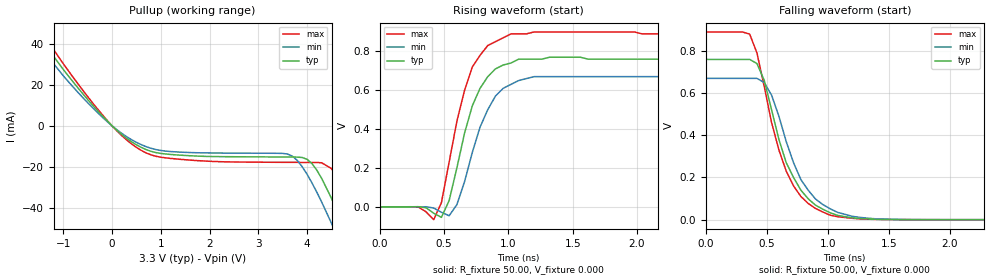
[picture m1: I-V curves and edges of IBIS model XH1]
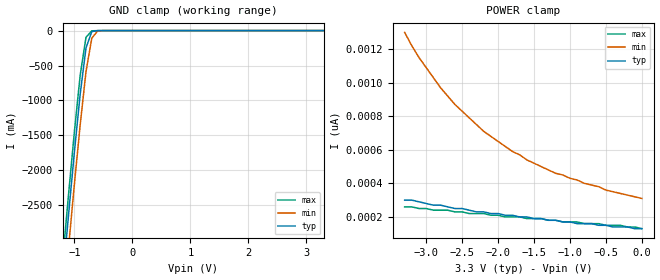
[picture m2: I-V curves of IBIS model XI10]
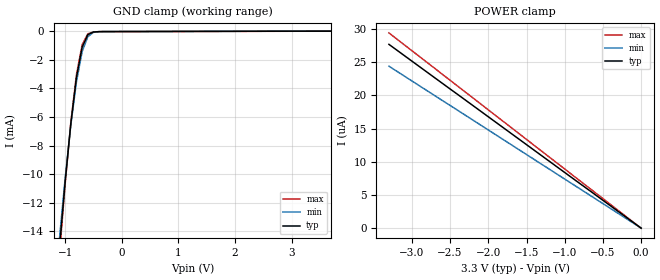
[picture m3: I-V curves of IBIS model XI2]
|   * 9db401d.ibs * IBIS 2.1 Model file
| Rev History
| Rev No.   Description
| 1.0   Initial release
| 1.1   Updated Parasitic Parameters,
|   Input and output C_comp min / Max tightened + Added pin RLC
| 1.2   Update parameters   August 8, 2005
| 1.3   Update XH1, XIO3 Jan. 06, 2010
| 1.4   Add Vmeas, Vref, Ref. May 2010 lp
[IBIS Ver]   2.1
[Comment char]  |_char
[File name]   9db401d.ibs
[Date]   May 10, 2010
[File Rev]   1.4
[Source]   Originated at Integrated Circuit Systems, Inc.
[Disclaimer] (C) Copyright Integrated Circuit Systems, Inc. 2004
   All rights reserved
ICS hereby grants the user of this IBIS model a non-exclusive,
nontransferable license to use this IBIS model under the following terms.
Before using this IBIS model, the user should read this license.
If the user does not accept these terms,  the IBIS model should be
returned to ICS within 30 days.
   The user is granted this license only to use the IBIS model and
is not granted rights to sell, load, rent, lease or license the IBIS
model in whole or in part, or in modified form to anyone other than
user. User may modify the IBIS model to suit its specific
applications but rights to derivative works and such modifications
shall belong to ICS.
   This IBIS model is provided on an "AS IS" basis and ICS makes
absolutely no warranty with respect to the information contained
herein. ICS DISCLAIMS AND CUSTOMER WAIVES ALL WARRANTIES, EXPRESS
OR IMPLIED, INCLUDING WARRANTIES OF MERCHANTABILITY OR FITNESS FOR
A PARTICULAR PURPOSE. The entire risk as to quality and performance
is with the Customer. ACCORDINGLY, IN NO EVENT SHALL THE COMPANY BE
LIABLE FOR ANY DAMAGES, WHETHER IN CONTRACT OR TORT,INCLUDING ANY
LOST PROFITS OR OTHER INCIDENTAL, CONSEQUENTIAL, EXEMPLARY, OR
PUNITIVE DAMAGES ARISING OUT OF THE USE OR APPLICATION OF THE IBIS
model provided in this package. Further, ICS reserves the right to
make changes without notice to any product herein to improve
reliability, function, or design. ICS does not convey any license
under patent rights or any other intellectual property rights,
including those of third parties.
   ICS is not obligated to provide maintenance or support
for the licensed IBIS model.
|   COMPONENT: ICS9db401d
[Component]   ICS9db401d
[Manufacturer]  ICS
[Package]
| variable   typ   min   max
R_pkg   81.1m   62.2m   100.0m
L_pkg   6.7nH   4.9nH   8.5nH
C_pkg   0.53pF  0.21pF  0.85pF
[Pin]   signal_name   model_name   R_pin   L_pin   C_pin
  1   VDD   POWER   90.5m   4.72nH  0.585pF
  2   SRC_IN   XI4   91.3m   4.11nH  0.57pF
  3   SRC_IN#   XI4   93.6m   3.68nH  0.433pF
  4   GND   GND   39.9m   2.61nH  0.44pF
  5   VDD   POWER   92.1m   3.14nH  0.318pF
  6   DIF_1   XH1   78m   2.79nH  0.286pF
  7   DIF_1#   XH1   70.5m   2.62nH  0.272pF
  8   OE_1(OE_1#)   XI23   39.8m   2.27nH  0.311pF
  9   DIF_2   XH1   74.7m   2.7nH   0.279pF
 10   DIF_2#   XH1   86m   3nH   0.294pF
 11   VDD   POWER   53.2m   2.8nH   0.356pF
 12   BYPASS#/PLL   XI23   97.1m   3.84nH  0.432pF
 13   SCLK   XI10   93.6m   4.23nH  0.58pF
 14   SDATA   XIO3   91.4m   4.77nH  0.595pF
 15   PD#(PD)   XI2   91.2m   4.76nH  0.592pF
 16   SRC_STOP#(SRC_STOP)   XI23   93.7m   4.22nH  0.579pF
 17   HIGH_BW#   XI23   97.8m   3.84nH  0.434pF
 18   VDD   POWER   95.6m   3.34nH  0.295pF
 19   DIF_5#   XH1   82.6m   2.93nH  0.285pF
 20   DIF_5   XH1   73.4m   2.67nH  0.277pF
 21   OE_6(OE_6#)   XI23   40m   2.26nH  0.308pF
 22   DIF_6#   XH1   70.8m   2.62nH  0.273pF
 23   DIF_6   XH1   80.8m   2.86nH  0.293pF
 24   VDD   POWER   52.4m   2.73nH  0.378pF
 25   OE_INV#(OE_INV)   XI24   40.3m   2.63nH  0.436pF
 26   IREF   NC   95.1m   3.75nH  0.434pF
 27   GNDA   GND   56.9m   3.8nH   0.63pF
 28   VDDA   POWER   58m   4.46nH  0.642pF
|* Either 3.3V or 2.5V
|** All model are simulated with typical corner process
[Diff Pin]   inv_pin   vdiff   tdelay_typ
2   3   NA   NA
6   7   NA   NA
9   10   NA   NA
20   19   NA   NA
23   22   NA   NA
| Models and submodels in the file (7): XH1 (Open_source), XI10 (Input), XI2 (Input), XI23 (Input), XI24 (Input), XI4 (Input), XIO3 (I/O_open_drain)
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|   Model XH1
[Model]   XH1
Model_type   Open_source
Polarity   Inverting
Vmeas = 0.35V
Cref =   2.00pF
Rref =  500
Vref =   0.0V
C_comp   3.40pF   2.85pF   3.95pF
[Temperature Range]   25.00   70.00   0.000
[Voltage Range]   3.30V   3.00V   3.70V
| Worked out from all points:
|   slope of the pullup table from 0 to 0.495 V, typ, clamps not added: 53.7 ohm
|   rising waveform, R_fixture 50.00, V_fixture 0.000: 20-80 % time 196ps typ, 209ps min, 191ps max; typ from 0 V to 0.76 V
|   falling waveform, R_fixture 50.00, V_fixture 0.000: 20-80 % time 266ps typ, 276ps min, 255ps max; typ from 0.76 V to 0 V
[Pullup]
| voltage   I(typ)   I(min)   I(max)
-3.3V     120mA      110mA      120mA
-1.9V     57.97mA    52.49mA    62.98mA
-1.5V     43.73mA    39.31mA    47.78mA
-100mV    2.37mA     2.07mA     2.66mA
700mV     -11.65mA   -10.21mA   -13.27mA
3.6V      -15.27mA   -13.83mA   -17.88mA
4V        -16.4mA    -23.77mA   -17.93mA
4.3V      -25.83mA   -37.4mA    -18.11mA
4.5V      -35.53mA   -47.74mA   -20.97mA
4.7V      -46.5mA    -58.63mA   -28.65mA
5.1V      -70.24mA   -81.19mA   -50.61mA
6.6V      -160mA     -170mA     -150mA
[Ramp]
| variable   typ   min   max
dV/dt_r   0.46/0.20n   0.40/0.21n   0.53/0.19n
dV/dt_f   0.45/0.26n   0.40/0.27n   0.53/0.25n
R_load = 50.00
[Rising Waveform]
R_fixture = 50.00
V_fixture = 0.000
V_fixture_min = 0.000
V_fixture_max = 0.000
| time   V(typ)   V(min)   V(max)
0s        -370nV     -380nV     -340nV
300ps     550uV      230uV      -1.44mV
420ps     -32.86mV   -6.35mV    -66.34mV
480ps     -54.44mV   -28.27mV   21.55mV
540ps     32.24mV    -46.01mV   230mV
600ps     200mV      10.91mV    440mV
720ps     520mV      280mV      720mV
840ps     670mV      500mV      830mV
1.02ns    740mV      630mV      890mV
3ns       760mV      670mV      890mV
[Falling Waveform]
R_fixture = 50.00
V_fixture = 0.000
V_fixture_min = 0.000
V_fixture_max = 0.000
| time   V(typ)   V(min)   V(max)
0s        760mV      670mV      890mV
360ps     760mV      670mV      880mV
420ps     740mV      670mV      790mV
480ps     660mV      650mV      630mV
540ps     520mV      590mV      460mV
660ps     270mV      370mV      230mV
780ps     140mV      190mV      110mV
900ps     68.75mV    97.98mV    52.94mV
1.38ns    2.27mV     4.59mV     1.49mV
3ns       -13.74uV   -37.6uV    -15.05uV
|   Model XI10
[Model]   XI10
Model_type   Input
Polarity   Inverting
Vinl =   0.80V
Vinh =   2.00V
C_comp   3.40pF   2.85pF   3.95pF
[Temperature Range]   27.00   70.00   0.000
[Voltage Range]   3.30V   3.00V   3.70V
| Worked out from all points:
|   GND clamp passes 1 mA (typ) near -0.60 V on its own axis
[GND_clamp]
| voltage   I(typ)   I(min)   I(max)
-3.3V     -24.05A    -24.49A    -23.79A
-1.2V     -3.55A     -4.02A     -3.26A
-1.1V     -2.63A     -3.1A      -2.34A
-1V       -1.74A     -2.2A      -1.45A
-900mV    -910mA     -1.35A     -640mA
-800mV    -250mA     -590mA     -96.82mA
-700mV    -14.58mA   -110mA     -3.87mA
-600mV    -880uA     -5.84mA    -450uA
-500mV    -88.5uA    -350uA     -45.09uA
3.3V      130pA      340pA      120pA
[POWER_clamp]
| voltage   I(typ)   I(min)   I(max)
-3.3V     300pA      1.3nA      260pA
-3.1V     290pA      1.15nA     250pA
-2.9V     270pA      1.03nA     240pA
-2.8V     270pA      970pA      240pA
-2.6V     250pA      870pA      230pA
-2.2V     230pA      710pA      220pA
-1.8V     210pA      590pA      200pA
-1.2V     180pA      460pA      180pA
-900mV    160pA      420pA      170pA
-500mV    150pA      360pA      150pA
-300mV    140pA      340pA      150pA
0V        130pA      310pA      130pA
|   Model XI2
[Model]   XI2
Model_type   Input
Polarity   Inverting
Vinl =   0.80V
Vinh =   2.00V
C_comp   3.40pF   2.85pF   3.95pF
[Temperature Range]   25.00   70.00   0.000
[Voltage Range]   3.30V   3.00V   3.70V
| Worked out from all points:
|   GND clamp passes 1 mA (typ) near -0.69 V on its own axis
[GND_clamp]
| voltage   I(typ)   I(min)   I(max)
-3.3V     -150mA     -140mA     -150mA
-1.1V     -15.17mA   -14.5mA    -15.62mA
-1V       -10.54mA   -10.3mA    -10.7mA
-900mV    -6.48mA    -6.58mA    -6.4mA
-800mV    -3.23mA    -3.54mA    -3.03mA
-700mV    -1.13mA    -1.43mA    -950uA
-600mV    -250uA     -390uA     -190uA
-500mV    -58.48uA   -85.04uA   -52.74uA
-400mV    -33.35uA   -32.48uA   -37.57uA
3.7V      170pA      5.18uA     140pA
[POWER_clamp]
| voltage   I(typ)   I(min)   I(max)
-3.3V     27.7uA     24.41uA    29.43uA
-3.2V     26.86uA    23.67uA    28.53uA
-2.7V     22.66uA    19.97uA    24.08uA
0V        140pA      2.62nA     140pA
